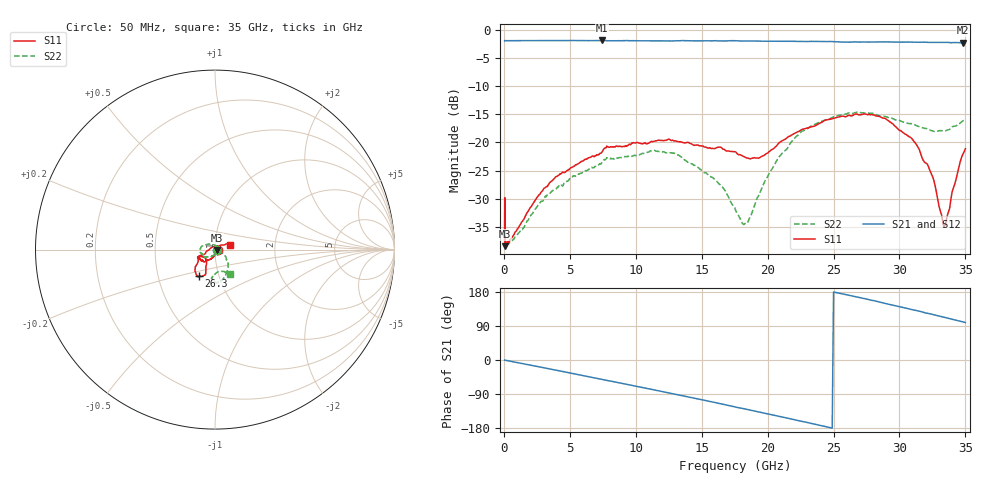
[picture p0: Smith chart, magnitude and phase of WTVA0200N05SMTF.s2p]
! 50 ohm 2-Port S-parameters measured by Modelithics Inc support@modelithics.com  Tampa, FL USA 813-866-6335 (February 2024)
! Smiths Interconnect,  2dB P/N: WTVA0200N05SMTF, Temperature: 25C
! Board: 10 mil Rogers 4350B, Mounting Pad Dimensions: Length: 15 mils, Width: 25 mils, Gap: 40 mils.
# Hz S MA R 50
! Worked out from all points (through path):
!   486 points, 50 MHz to 35 GHz, reference 50 ohm
!   highest |S21| = -1.92 dB at 7.45 GHz (marker M1); lowest = -2.3 dB at 34.8 GHz (marker M2)
!   group delay of S21, straight-line fit = 20.4 ps
!   lowest |S11| = -38.4 dB at 90 MHz (marker M3), VSWR 1.02, Z = 51.2 - j0.192 ohm
!   |S11| at or under -10 dB: start of sweep to end of sweep
!   |S22| runs from -38.2 to -14.6 dB; largest |S21 - S12| = 0.019
!   S11 on the Smith chart (normalised r, x): 50 MHz: 1.03, -0.00; 26.3 GHz: 0.80, -0.25; 35 GHz: 1.18, +0.07
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5e7  0.01429 -7.2  0.7967 -0.3  0.7968 -0.3  0.01319 -2.4
8e7  0.0138 -12.1  0.7978 -0.5  0.7969 -0.6  0.01354 -5.2
9e7  0.01205 -9.0  0.7977 -0.6  0.7974 -0.6  0.01229 -7.2
6.5e8  0.0146 -46.6  0.7979 -4.3  0.7977 -4.4  0.01361 -43.0
3.05e9  0.03934 -99.8  0.7974 -20.7  0.7972 -20.7  0.03154 -100.6
5.9e9  0.06813 -121.5  0.7992 -40.4  0.7991 -40.4  0.05356 -130.6
7.45e9  0.08253 -128.5  0.8015 -51.2  0.8015 -51.2  0.0666 -142.4
1.17e10  0.1047 -153.0  0.796 -81.1  0.7956 -81.0  0.08339 -177.8
1.31e10  0.1024 -156.3  0.7966 -90.9  0.7963 -90.9  0.07806 168.9
1.58e10  0.08883 -156.7  0.7947 -110.6  0.7947 -110.6  0.04909 141.9
1.76e10  0.08215 -150.5  0.7968 -124.5  0.7966 -124.2  0.02458 92.6
1.84e10  0.07291 -142.4  0.7929 -130.2  0.793 -130.0  0.01904 24.7
2.08e10  0.09734 -119.3  0.7886 -148.2  0.7881 -148.0  0.07244 -34.1
2.34e10  0.1385 -111.8  0.7865 -168.0  0.7869 -167.7  0.1414 -62.4
2.63e10  0.1722 -120.8  0.774 170.2  0.774 170.3  0.1818 -84.0
2.92e10  0.1544 -135.6  0.7777 147.1  0.7773 147.7  0.1656 -96.5
3.14e10  0.09105 -155.8  0.7717 129.6  0.7717 129.9  0.1391 -91.6
3.24e10  0.05327 -162.7  0.77 121.2  0.7698 121.6  0.1276 -85.2
3.34e10  0.01776 106.1  0.7718 112.9  0.7729 113.3  0.1269 -74.7
3.36e10  0.02185 69.7  0.7713 110.8  0.7705 111.8  0.1285 -71.2
3.48e10  0.07832 25.0  0.7644 100.7  0.7647 101.1  0.155 -58.5
3.5e10  0.08802 18.5  0.7653 98.9  0.7646 99.2  0.1606 -57.7
